// TwinCAT 3 PLC project Tutorial_01_UaServer_DataAccess
// ProgramVersion: 3.1.0.8
// libraries:
//   Tc2_Standard, * (Beckhoff Automation GmbH)
//   Tc2_System, * (Beckhoff Automation GmbH)
//   Tc3_Interfaces, * (Beckhoff Automation GmbH)
//   Tc3_Module, * (Beckhoff Automation GmbH)
// project tree:
//   / PlcTask.TcTTO
//   POUs/ FB_TEST.TcPOU, MAIN.TcPOU

CONFIGURATION Tutorial_01_UaServer_DataAccess
    RESOURCE PLC ON TwinCAT3
        TASK PlcTask(INTERVAL := T#10ms, PRIORITY := 20);
        PROGRAM MAIN WITH PlcTask : MAIN;
    END_RESOURCE
END_CONFIGURATION

// ---- POUs/MAIN.TcPOU
PROGRAM MAIN
VAR
	fbTest		: FB_TEST;
	{attribute 'OPC.UA.DA' := '1'}	
	fbTest2		: FB_TEST;
	
	(* Variables for input and output arguments of FB *)
	{attribute 'OPC.UA.DA' := '1'}
	value1		: INT;
	{attribute 'OPC.UA.DA' := '1'}
	value2		: INT;
	{attribute 'OPC.UA.DA' := '1'}
	nOutput1 	: INT;
	{attribute 'OPC.UA.DA' := '1'}
	nOutput2	: INT; 
END_VAR

fbTest2(
	nInput1 := value1,
	nInput2 := value2,
	nOutput1 => nOutput1,
	nOutput2 => nOutput2
);

END_PROGRAM

// ---- POUs/FB_TEST.TcPOU
FUNCTION_BLOCK FB_TEST
VAR_INPUT
	{attribute 'OPC.UA.DA' := '1'}
	nInput1		: INT; (*~ (OPC:1:available) *)
	nInput2		: INT;
END_VAR
VAR_OUTPUT
	{attribute 'OPC.UA.DA' := '1'}
	nOutput1 	: INT;
	nOutput2 	: INT;
END_VAR
VAR
	{attribute 'OPC.UA.DA' := '1'}
	nVariable 	: INT;
END_VAR

nVariable := nInput1 + nInput2;
nOutput1 := nVariable + nInput1;
nOutput2 := nVariable + nInput2;

END_FUNCTION_BLOCK
